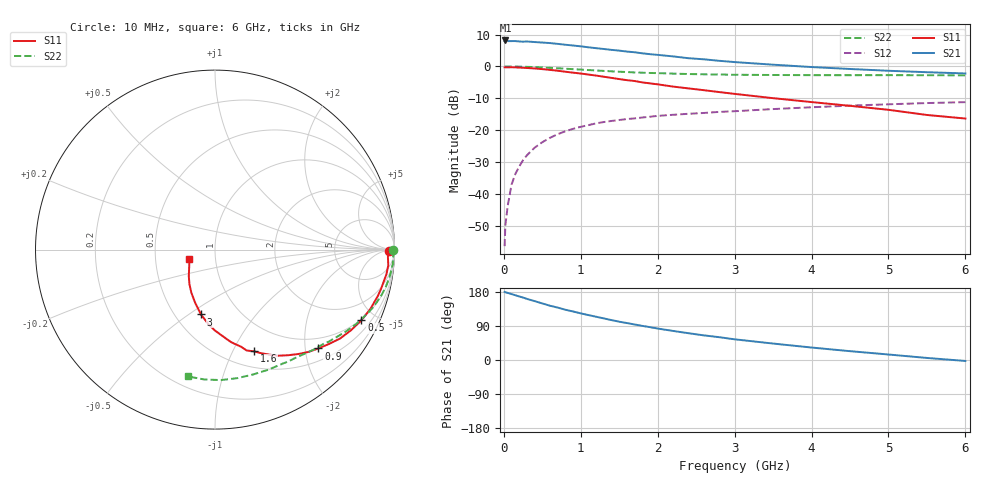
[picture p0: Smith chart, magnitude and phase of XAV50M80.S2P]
! SIEMENS Discrete & RF Semiconductors
! BFY180
! Si NPN RF Bipolar Junction Transistor in MICRO-X
! VCE = 0.5 V  IC = 0.8 mA
! Common Emitter S-Parameters:  May  1997
# GHz  S  MA  R  50
!  f  S11  S21  S12  S22
! GHz  MAG  ANG  MAG  ANG  MAG  ANG  MAG  ANG
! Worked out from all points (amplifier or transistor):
!   36 points, 10 MHz to 6 GHz, reference 50 ohm
!   highest |S21| = 8.1 dB at 20 MHz (marker M1)
!   |S21| within 3 dB of that: start of sweep to 1.417 GHz
!   unconditionally stable (mu >= 1): 2.531 GHz to end of sweep
!   at 250 MHz: K = 0.11, MSG = 18.6 dB, |S12| = -29.4 dB
!   at 1.4 GHz: K = 0.66, MSG = 11.2 dB, |S12| = -17.1 dB
!   at 6 GHz: K = 1.23, MAG = 1.6 dB, |S12| = -11.2 dB
!   S11 on the Smith chart (normalised r, x): 10 MHz: 57, -12; 500 MHz: 0.95, -4.16; 900 MHz: 0.76, -2.28; 1.6 GHz: 0.68, -1.21; 3 GHz: 0.67, -0.56; 6 GHz: 0.75, -0.08
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0.01  0.9667 -0.4  2.475 179.7  0.0015 92.5  0.9938 -0.2
0.02  0.9674 -1.0  2.553 178.7  0.0032 88.0  0.9953 -0.6
0.05  0.9642 -2.4  2.492 177.1  0.0064 86.4  0.9941 -1.6
0.1  0.9694 -5.2  2.495 174.0  0.0139 86.5  0.9927 -3.2
0.15  0.965 -8.2  2.497 170.9  0.0205 84.4  0.9938 -4.7
0.3  0.9433 -15.9  2.46 161.3  0.0401 78.5  0.9828 -9.3
0.5  0.9058 -25.8  2.367 149.3  0.0644 71.0  0.9624 -15.1
0.6  0.8807 -30.7  2.323 143.2  0.0755 67.9  0.9489 -17.8
0.8  0.824 -39.7  2.188 132.6  0.0956 61.1  0.9187 -23.0
0.9  0.7968 -43.7  2.126 128.0  0.1044 58.1  0.9044 -25.3
1.1  0.7442 -51.4  1.993 118.6  0.1195 52.8  0.8754 -29.6
1.3  0.6876 -59.3  1.875 109.7  0.1336 48.1  0.8487 -33.6
1.5  0.6319 -66.0  1.767 101.0  0.1438 44.0  0.8241 -37.3
1.6  0.6074 -69.0  1.708 97.5  0.1488 42.7  0.8153 -39.0
2  0.522 -80.3  1.516 83.0  0.1669 36.7  0.7832 -45.3
2.2  0.4814 -85.3  1.434 76.7  0.1736 33.7  0.7693 -48.4
2.6  0.4227 -94.3  1.291 65.0  0.1854 29.7  0.7501 -53.9
3  0.3698 -102.2  1.168 54.6  0.1975 25.6  0.7385 -59.4
3.5  0.3167 -110.4  1.063 43.4  0.2135 21.6  0.7321 -66.2
4.5  0.24 -126.4  0.91 23.3  0.2418 12.4  0.7269 -80.1
5.5  0.1724 -146.5  0.81 5.4  0.2653 3.4  0.7262 -94.7
6  0.1516 -160.3  0.774 -2.5  0.2744 -1.4  0.7223 -101.9
